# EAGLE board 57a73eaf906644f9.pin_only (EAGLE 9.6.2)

Size 33.28 x 17.76 mm. Coordinates in mm from the lower left corner, seen from the top.
Outline: 0,0.12 0,6.54 arc-90 10.38,17.76 23.79,17.71 arc-90 33.25,6.64 33.25,0.12
Outline: 0,0 33.25,0
Copper layers (1*16): Top 0.035mm / dielectric 1.5mm / Bottom 0.035mm
Design rules "default *": minimum track width 12mil, minimum drill 20mil, track to track 12mil, track to pad 12mil, pad to pad 30mil, via to via 12mil, smd to smd 0mil, copper to edge 15mil, drill to drill 8mil, minimum pad ring 10mil, minimum via ring 8mil, stop-mask expansion 4mil, vias tented up to drill 0mil, thermal gap 10mil

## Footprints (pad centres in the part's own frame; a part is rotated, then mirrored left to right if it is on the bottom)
1X01 = drill 1.016 pad 1.93 octagon: 1 0,0
C025-025X050 = drill 0.813 pad 1.676 octagon: 1 -1.27,0; 2 1.27,0
E2,5-5 = drill 0.813 pad 1.6: + -1.27,0 | drill 0.813 pad 1.6 octagon: - 1.27,0
DO41-7 = drill 1.118 pad 1.93: A 4,0; C -4,0
DIL08 = drill 0.813 long: 1 -3.81,-3.81; 2 -1.27,-3.81; 3 1.27,-3.81; 4 3.81,-3.81; 5 3.81,3.81; 6 1.27,3.81; 7 -1.27,3.81; 8 -3.81,3.81
6000 = drill 1.2 pad 2.184: 1 -2.5,0; 2 2.5,0
0204/5 = drill 0.813 pad 1.676 octagon: 1 -2.54,0; 2 2.54,0
PN87520 = drill 0.95 long: 1 -3.5,2.71; 2 -1,2.71; 3 1,2.71; 4 3.5,2.71 | drill 2.286: P$1 -6.604,0; P$2 6.604,0

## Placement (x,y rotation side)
+  [1X01]  1.99,1.78 0 top
-  [1X01]  31.35,1.85 0 top
C1  0.1uF  [C025-025X050]  5.9,1.37 0 top
C2  0.1uF  [C025-025X050]  10.62,1.4 180 top
C3  220uF  [E2,5-5]  6.02,12.93 180 top
C4  220uF  [E2,5-5]  29.7,5.56 270 top
D1  1N5817  [DO41-7]  25.53,5.89 270 top
IC1  LT1302  [DIL08]  18.65,5.61 90 top
L1  L  [6000]  9.69,6.97 270 top
R1  49.9K  [0204/5]  4.65,6.73 90 top
R2  75K  [0204/5]  2.13,7.6 270 top
R3  49.9K  [0204/5]  29.28,10.53 145 top
R4  75K  [0204/5]  28.68,13.28 140 top
R5  3.3k  [0204/5]  18.75,5.59 90 top
X1  [PN87520]  16.67,15.44 180 top

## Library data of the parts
+ - = pinhead-ez
C1-C4 D1 IC1 L1 R1-R5 = adafruit
X1 = con-berg

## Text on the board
tPlace: + | -
bPlace: v3 | LT1302 | adafruit! | MintyBoost!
